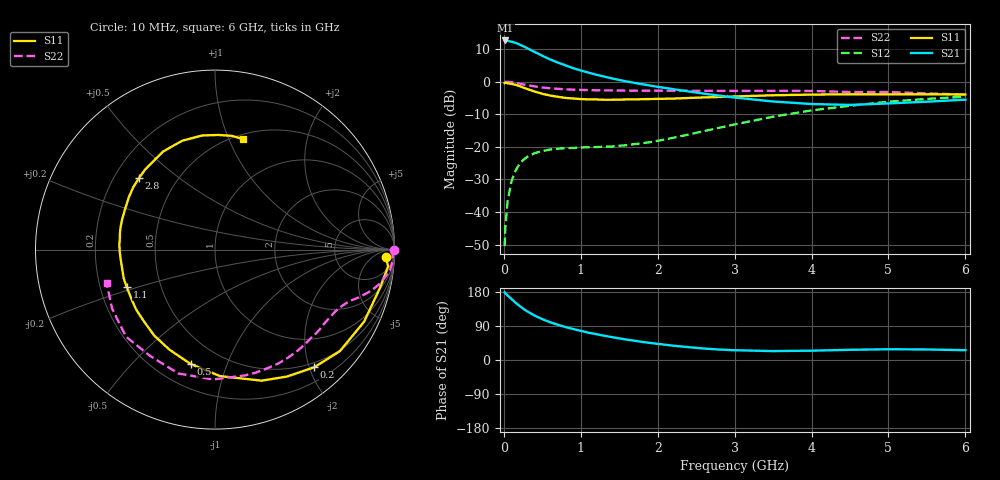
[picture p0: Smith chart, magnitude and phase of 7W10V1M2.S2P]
! Infineon Technologies  Discrete & RF Semiconductors
! BFS17W
! Si NPN RF Bipolar Junction Transistor in SOT323
! VCE = 10 V  IC = 1.2 mA
! Common Emitter S-Parameters:  August  1999
# GHz  S  MA  R  50
!  f  S11  S21  S12  S22
! GHz  MAG  ANG  MAG  ANG  MAG  ANG  MAG  ANG
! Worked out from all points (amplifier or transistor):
!   36 points, 10 MHz to 6 GHz, reference 50 ohm
!   highest |S21| = 12.6 dB at 20 MHz (marker M1)
!   |S21| within 3 dB of that: start of sweep to 355 MHz
!   unconditionally stable (mu >= 1): 1.03 GHz to 2.954 GHz; 4.187 GHz to end of sweep
!   at 250 MHz: K = 0.27, MSG = 17.5 dB, |S12| = -24.1 dB
!   at 1.4 GHz: K = 1.24, MAG = 7.5 dB, |S12| = -19.9 dB
!   at 6 GHz: K = 1.08, MAG = -2.2 dB, |S12| = -4.6 dB
!   S11 on the Smith chart (normalised r, x): 10 MHz: 23, -21; 200 MHz: 0.42, -2.08; 500 MHz: 0.34, -0.75; 1.1 GHz: 0.31, -0.18; 2.8 GHz: 0.30, +0.37; 6 GHz: 0.55, +1.13
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0.01  0.9536 -2.5  4.261 178.7  0.003 83.0  0.9999 -0.2
0.02  0.969 -5.6  4.284 176.1  0.006 89.9  0.9892 -1.4
0.05  0.9433 -13.2  4.231 170.1  0.015 83.4  0.9922 -3.4
0.1  0.9227 -25.8  4.092 160.9  0.0299 75.8  0.9816 -6.7
0.15  0.8969 -39.1  3.948 151.5  0.0427 68.3  0.9576 -9.5
0.2  0.8574 -49.9  3.729 143.3  0.0539 63.3  0.9345 -11.9
0.25  0.8133 -60.4  3.501 135.7  0.0626 57.5  0.9088 -14.0
0.3  0.7751 -70.4  3.27 128.9  0.0699 53.5  0.8862 -15.6
0.4  0.7053 -87.7  2.852 117.1  0.0801 46.8  0.8455 -18.3
0.5  0.6518 -102.0  2.497 107.8  0.0863 42.5  0.8138 -20.2
0.6  0.6124 -114.6  2.196 99.8  0.091 39.7  0.7923 -21.9
0.7  0.5867 -125.2  1.968 93.1  0.0937 38.5  0.7766 -23.6
0.8  0.5631 -134.5  1.781 87.0  0.0956 37.9  0.7635 -25.4
1.1  0.5344 -156.9  1.377 72.1  0.0989 40.0  0.7421 -30.9
1.6  0.5336 177.1  1.004 53.7  0.1063 50.3  0.728 -41.4
2.2  0.5502 155.1  0.768 37.8  0.1376 64.8  0.7267 -55.9
2.8  0.5818 136.6  0.61 27.6  0.1961 71.6  0.7222 -71.7
3.5  0.6183 118.0  0.496 23.5  0.2902 70.1  0.7236 -90.8
4  0.6336 106.7  0.454 24.6  0.3626 64.8  0.7198 -106.4
4.5  0.6397 96.4  0.44 26.9  0.4263 58.1  0.6942 -121.4
5.5  0.6408 81.5  0.493 27.8  0.5438 44.0  0.6609 -150.2
6  0.635 75.9  0.53 25.9  0.5886 37.2  0.6315 -163.1
